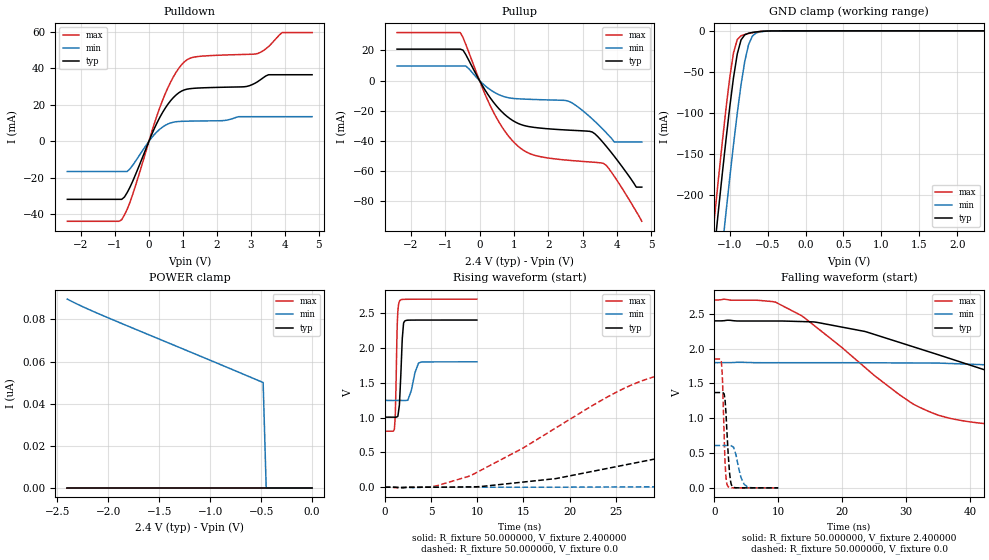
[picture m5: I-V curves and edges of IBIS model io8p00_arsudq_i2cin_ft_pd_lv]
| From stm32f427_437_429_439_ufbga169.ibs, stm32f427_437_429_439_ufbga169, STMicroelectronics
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|   Model io8p00_arsudq_i2cin_ft_pd_lv
[Model]  io8p00_arsudq_i2cin_ft_pd_lv
Model_type I/O
Polarity   Non-Inverting
Enable   Active-Low
Vinl =   0.720000V
Vinh =   1.680000V
Vmeas =  1.200000V
Cref =   50.000000pF
Rref =   100.000000M
Vref =   0.0V
C_comp   2.226900pF   2.174000pF   2.332300pF
[Temperature Range]   25.000000   0.125000k   -40.000000
[Pullup Reference]   2.400000V   1.800000V   2.700000V
[Pulldown Reference]   0.0V   0.0V   0.0V
[POWER Clamp Reference]   2.400000V   1.800000V   2.700000V
[GND Clamp Reference]   0.0V   0.0V   0.0V
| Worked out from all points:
|   slope of the pulldown table from 0 to 0.36 V, typ, clamps not added: 25 ohm
|   slope of the pullup table from 0 to 0.36 V, typ, clamps not added: 27.7 ohm
|   GND clamp passes 1 mA (typ) near -0.62 V on its own axis
|   rising waveform, R_fixture 50.000000, V_fixture 2.400000: 20-80 % time 270ps typ, 605ps min, 184ps max; typ from 1 V to 2.4 V
|   rising waveform, R_fixture 50.000000, V_fixture 0.0: 20-80 % time 32.4ns typ, 81.1ns min, 14.7ns max; typ from 0 V to 1.37 V
|   falling waveform, R_fixture 50.000000, V_fixture 2.400000: 20-80 % time 29.2ns typ, 72.1ns min, 15.7ns max; typ from 2.4 V to 1 V
|   falling waveform, R_fixture 50.000000, V_fixture 0.0: 20-80 % time 523ps typ, 972ps min, 382ps max; typ from 1.37 V to 0 V
[Pulldown]
|Voltage   I(typ)   I(min)   I(max)
-2.4V     -31.73mA   -16.51mA   -43.74mA
-800mV    -31.73mA   -16.51mA   -42.87mA
-480mV    -21.98mA   -13.17mA   -29.2mA
80mV      3.63mA     1.966mA    5.014mA
480mV     18.15mA    8.738mA    26.02mA
800mV     25.38mA    10.72mA    37.77mA
1.12V     28.53mA    11.02mA    44.6mA
2.8V      29.84mA    13.49mA    47.53mA
3.2V      32.65mA    13.49mA    48.04mA
3.52V     36.42mA    13.49mA    51.83mA
3.92V     36.42mA    13.49mA    59.49mA
4.8V      36.42mA    13.49mA    59.49mA
[Pullup]
|Voltage   I(typ)   I(min)   I(max)
-2.4V     20.89mA    9.659mA    31.9mA
-560mV    20.89mA    9.659mA    31.9mA
-400mV    17.28mA    9.659mA    24.07mA
320mV     -11.75mA   -6.207mA   -17.08mA
960mV     -26.47mA   -11.82mA   -40.02mA
1.52V     -30.88mA   -12.51mA   -49.05mA
2.56V     -32.88mA   -13.48mA   -52.9mA
3.28V     -34.19mA   -25.52mA   -54.18mA
3.6V      -41.31mA   -32.62mA   -54.97mA
3.92V     -50.33mA   -40.8mA    -63.63mA
4.56V     -70.8mA    -40.8mA    -87.07mA
4.72V     -70.8mA    -40.8mA    -93.5mA
[GND_clamp]
|Voltage   I(typ)   I(min)   I(max)
-2.4V     -1.424A    -1.508A    -1.393A
-1.25V    -311.2mA   -401.9mA   -273.3mA
-1.2V     -265.4mA   -356.1mA   -227.2mA
-1.15V    -220.4mA   -310.8mA   -181.9mA
-1.1V     -176.3mA   -266.2mA   -137.9mA
-1.05V    -133.8mA   -222.5mA   -95.87mA
-950mV    -57.3mA    -138.9mA   -26.99mA
-900mV    -28.28mA   -100.4mA   -10.6mA
-850mV    -11.02mA   -65.54mA   -5.972mA
-750mV    -2.846mA   -16.51mA   -3.192mA
-600mV    -761.3uA   -1.173mA   -751.9uA
2.35V     58.09uA    37.92uA    67.25uA
[POWER_clamp]
|Voltage   I(typ)   I(min)   I(max)
-2.4V     0A         89.62nA    0A
-2.04V    0A         81.57nA    0A
-480mV    0A         50.01nA    0A
-450mV    0A         0A         0A
0V        0A         0A         0A
[Ramp]
| variable   typ   min   max
dV/dt_r  0.82206/32.39263n   0.36163/82.84955n   1.11048/14.72522n
dV/dt_f  0.83772/29.27444n   0.32730/74.37981n   1.13679/15.72746n
R_load = 50.000000
[Rising Waveform]
R_fixture= 50.000000
V_fixture= 2.400000
V_fixture_min= 1.800000
V_fixture_max= 2.700000
|time   V(typ)   V(min)   V(max)
0s        1.005V     1.245V     804.1mV
1.041ns   1.005V     1.245V     838.7mV
1.141ns   1.005V     1.246V     1.059V
1.381ns   1.014V     1.246V     2.443V
1.642ns   1.343V     1.246V     2.679V
1.902ns   2.146V     1.245V     2.695V
2.162ns   2.385V     1.244V     2.696V
2.503ns   2.397V     1.251V     2.697V
3.664ns   2.399V     1.784V     2.698V
9.97ns    2.399V     1.799V     2.699V
[Rising Waveform]
R_fixture= 50.000000
V_fixture= 0.0
V_fixture_min= 0.0
V_fixture_max= 0.0
|time   V(typ)   V(min)   V(max)
0s        10.14nV    256.5nV    17.63nV
5.005ns   -210uV     -66.11uV   7.502mV
9.009ns   4.963mV    -58.33uV   153mV
18.52ns   123.7mV    457uV      851.4mV
28.53ns   386.1mV    5.779mV    1.558V
41.04ns   747.8mV    35.82mV    1.783V
66.07ns   1.243V     124.3mV    1.842V
80.58ns   1.318V     196.5mV    1.848V
148.1ns   1.368V     492.4mV    1.851V
249.2ns   1.369V     608.5mV    1.851V
[Falling Waveform]
R_fixture= 50.000000
V_fixture= 2.400000
V_fixture_min= 1.800000
V_fixture_max= 2.700000
|time   V(typ)   V(min)   V(max)
0s        2.399V     1.799V     2.699V
9.51ns    2.397V     1.798V     2.67V
16.02ns   2.378V     1.798V     2.302V
31.03ns   2.029V     1.794V     1.207V
36.54ns   1.867V     1.788V     1.006V
44.04ns   1.642V     1.763V     907.9mV
59.06ns   1.254V     1.714V     845mV
87.09ns   1.072V     1.556V     815.7mV
137.1ns   1.019V     1.351V     805.4mV
249.2ns   1.005V     1.245V     804.1mV
[Falling Waveform]
R_fixture= 50.000000
V_fixture= 0.0
V_fixture_min= 0.0
V_fixture_max= 0.0
|time   V(typ)   V(min)   V(max)
0s        1.369V     608.5mV    1.851V
1.061ns   1.369V     608.4mV    1.819V
1.261ns   1.369V     608.4mV    1.52V
1.662ns   1.254V     608.2mV    357.6mV
1.842ns   997mV      607.9mV    111.2mV
2.042ns   649.5mV    607.8mV    32.02mV
2.482ns   114.9mV    609.9mV    2.415mV
2.843ns   16.57mV    592.8mV    431.3uV
4.645ns   36.16uV    50.72mV    25.3uV
9.97ns    10.14nV    256.5nV    17.63nV
